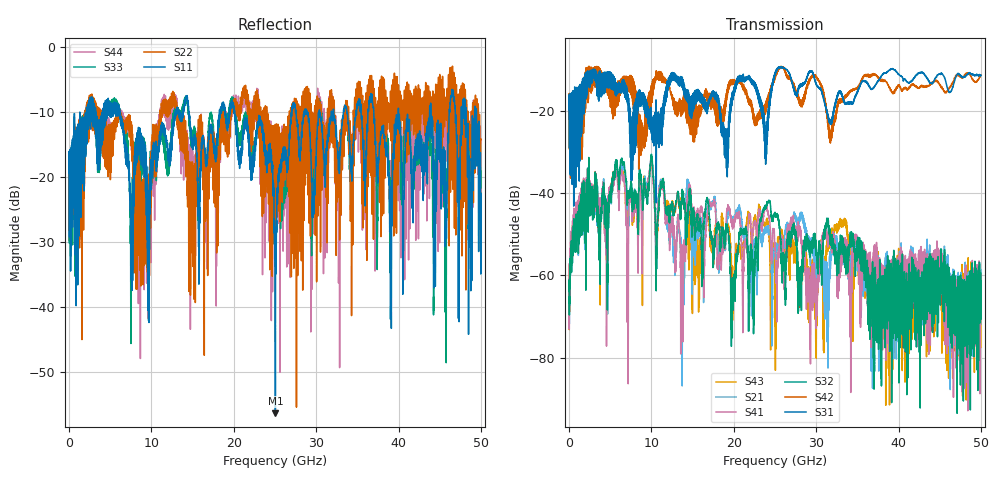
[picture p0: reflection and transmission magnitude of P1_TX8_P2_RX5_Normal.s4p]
!Keysight Technologies,N5225B,MY57041031,A.13.20.10
!Date: Friday, May 31, 2019 11:35:40
!Correction: S11(Full 4 Port(1,2,3,4))
!S12(Full 4 Port(1,2,3,4))
!S13(Full 4 Port(1,2,3,4))
!S14(Full 4 Port(1,2,3,4))
!S21(Full 4 Port(1,2,3,4))
!S22(Full 4 Port(1,2,3,4))
!S23(Full 4 Port(1,2,3,4))
!S24(Full 4 Port(1,2,3,4))
!S31(Full 4 Port(1,2,3,4))
!S32(Full 4 Port(1,2,3,4))
!S33(Full 4 Port(1,2,3,4))
!S34(Full 4 Port(1,2,3,4))
!S41(Full 4 Port(1,2,3,4))
!S42(Full 4 Port(1,2,3,4))
!S43(Full 4 Port(1,2,3,4))
!S44(Full 4 Port(1,2,3,4))
!S4P File: Measurements: <S11,S12,S13,S14>,
!<S21,S22,S23,S24>,
!<S31,S32,S33,S34>,
!<S41,S42,S43,S44>:
# Hz S  dB  R 50.0
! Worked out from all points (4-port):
!   5000 points, 10 MHz to 50 GHz, reference 50 ohm
!   strongest paths, dB at 10 MHz, 12.51 GHz, 25.01 GHz, 37.51 GHz, 50 GHz:
!     S31: -19.6, -10.7, -11.0, -12.6, -11.3
!     S42: -19.4, -16.9, -11.8, -11.8, -11.2
!     S32: -63.9, -42.8, -44.8, -68.9, -59.4
!     S41: -57.2, -47.8, -52.0, -57.4, -66.4
!     S21: -67.2, -48.0, -54.4, -56.9, -69.0
!     S43: -57.6, -42.7, -71.3, -56.0, -69.2
!   lowest |S11| = -56.3 dB at 25.05 GHz (marker M1), VSWR 1.00, Z = 49.8 - j0.0244 ohm
!   |S11| at or under -10 dB: 6.186 GHz to 12.89 GHz (6.703 GHz wide, 70.3 % of centre); 20.1 GHz to 26.99 GHz (6.893 GHz wide, 29.3 % of centre); 40 GHz to 43.77 GHz (3.764 GHz wide, 8.99 % of centre)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
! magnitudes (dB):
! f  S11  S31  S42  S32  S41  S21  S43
! 10 MHz  -19.4  -19.6  -19.4  -63.9  -57.2  -67.2  -57.6
! 6.49 GHz  -11.8  -12.5  -15.1  -32.8  -36.7  -34.1  -35.5
! 13.78 GHz  -10.1  -14.3  -20.6  -39.5  -57.6  -64.2  -40.1
! 14.44 GHz  -8.9  -15.2  -20.1  -45.9  -41.0  -37.9  -48.4
! 19.86 GHz  -8.8  -16.0  -12.8  -61.8  -48.7  -48.1  -70.9
! 25.05 GHz  -56.3  -10.5  -11.7  -45.6  -54.8  -53.3  -83.1
! 50 GHz  -22.5  -11.3  -11.2  -59.4  -66.4  -69.0  -69.2
